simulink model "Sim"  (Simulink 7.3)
settings: Solver=ode45  StartTime=0.0  StopTime=30  MaxStep=0.01  RelTol=1e-3
InitFcn:
  | r2d=180/pi;
  | [Avn,Bvn,Cvn,Dvn]= Vehi_20flx;              % Load Nomin Inters. Stiff Vehi
  | [Avr,Bvr,Cvr,Dvr]= Vehi_20rif;              % Load Hard Interst. Stiff Vehi
  | [Avs,Bvs,Cvs,Dvs]= Vehi_20sif;              % Load Soft Interst. Stiff Vehi
  | [Aa,Ba,Ca,Da]= actuator;                    % Load Actuator system
  | 
  | zn=0.02; wn=7.4; zd=0.2; wd=7;              % Filter-1
  | zn2=0.015; wn2=16.8; zd2=0.2; wd2=16;       % Filter-2
  | %[Af,Bf,Cf,Df]= linmod('Actor'); sysf= SS(Af,Bf,Cf,Df);
  | Iy=2.163e8; T=2847083; l=113.6;
  | om=0.145*6.28; wf=9;
  | Kp=om^2*Iy/(l*T); Kr=2*0.85*om*Iy/(l*T);
  | 
  | Av2=Avs; Bv2=Bvs; Cv2=Cvs; Dv2=Dvs;       % Use the Nominal in the Simulat
StopFcn:
  | Pl
undefined symbols (not defined in the file or in its folder): Aa, Ba, Ca, Da

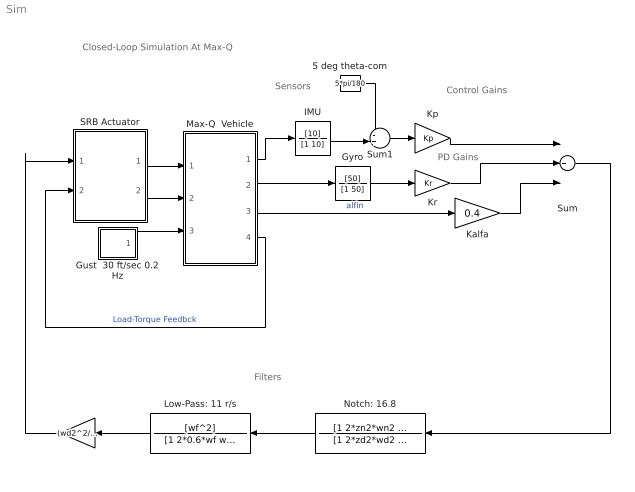
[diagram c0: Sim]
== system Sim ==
  note: Sensors
  note: PD Gains
  note: Filters
  note: Closed-Loop Simulation At Max-Q
  note: Control Gains
  "  " : Gain  Gain=(wd2^2/wn2^2)  ParameterDataType=sfix(16)  ParameterScaling=2^0  OutDataType=sfix(16)  OutScaling=2^0
  5 deg theta-com : Constant  Value=5*pi/180  OutDataType=sfix(16)  OutScaling=2^0
  Gust  30 ft/sec 0.2 Hz : Subsystem
  Gyro : TransferFcn  Numerator=[50]  Denominator=[1 50]
  IMU : TransferFcn  Numerator=[10]  Denominator=[1 10]
  Kalfa : Gain  Gain=0.4  ParameterDataType=sfix(16)  ParameterScaling=2^0  OutDataType=sfix(16)  OutScaling=2^0
  Kp : Gain  Gain=Kp  ParameterDataType=sfix(16)  ParameterScaling=2^0  OutDataType=sfix(16)  OutScaling=2^0
  Kr : Gain  Gain=Kr  ParameterDataType=sfix(16)  ParameterScaling=2^0  OutDataType=sfix(16)  OutScaling=2^0
  Low-Pass: 11 r/s : TransferFcn  Numerator=[wf^2]  Denominator=[1 2*0.6*wf wf^2]
  Max-Q  Vehicle : Subsystem
  Notch: 16.8 : TransferFcn  Numerator=[1 2*zn2*wn2 wn2^2]  Denominator=[1 2*zd2*wd2 wd2^2]
  SRB Actuator : Subsystem
  Sum : Sum  Inputs=+++  OutDataType=sfix(16)  OutScaling=2^0
  Sum1 : Sum  Inputs=-+|  OutDataType=sfix(16)  OutScaling=2^0
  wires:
  SRB Actuator/1(delto) -> Max-Q  Vehicle/1(delta)
  SRB Actuator/2(delt-dd) -> Max-Q  Vehicle/2(delt-dd)
  Max-Q  Vehicle/4(TL) -> SRB Actuator/2(Ld-Tq)  "Load-Torque Feedbck"
  Max-Q  Vehicle/3(alflex) -> Kalfa/1  "alfin"
  Kp/1 -> Sum/1
  Kr/1 -> Sum/2
  Max-Q  Vehicle/1(Theta) -> IMU/1
  Max-Q  Vehicle/2(q-flx) -> Gyro/1
  Sum/1 -> Notch: 16.8/1
  Gyro/1 -> Kr/1
  Low-Pass: 11 r/s/1 -> "  "/1
  Gust  30 ft/sec 0.2 Hz/1(Vgust) -> Max-Q  Vehicle/3(Gust)
  IMU/1 -> Sum1/2
  Sum1/1 -> Kp/1
  Kalfa/1 -> Sum/3
  Notch: 16.8/1 -> Low-Pass: 11 r/s/1
  "  "/1 -> SRB Actuator/1(delti)
  5 deg theta-com/1 -> Sum1/1

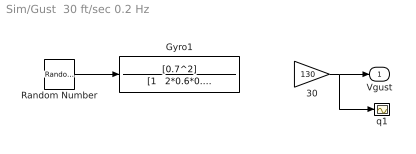
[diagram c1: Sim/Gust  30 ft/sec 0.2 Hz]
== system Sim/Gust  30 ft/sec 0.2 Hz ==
  30 : Gain  Gain=130  ParameterDataType=sfix(16)  ParameterScaling=2^0  OutDataType=sfix(16)  OutScaling=2^0
  Gyro1 : TransferFcn  Numerator=[0.7^2]  Denominator="[1   2*0.6*0.7   0.7^2]"
  Random Number : RandomNumber  Seed=-2  SampleTime=0
  q1 : Scope
  Vgust : Outport  OutDataType=sfix(16)  OutScaling=2^0
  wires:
  Random Number/1 -> Gyro1/1
  30/1 -> Vgust/1, q1/1

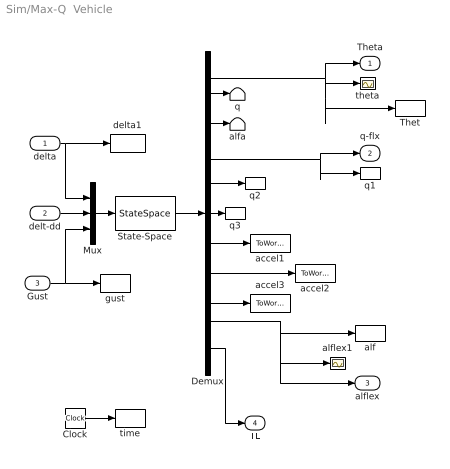
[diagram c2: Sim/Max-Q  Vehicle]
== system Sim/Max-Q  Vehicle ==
  delta : Inport  OutDataType=sfix(16)  OutScaling=2^0
  delt-dd : Inport  Port=2  OutDataType=sfix(16)  OutScaling=2^0
  Gust : Inport  Port=3  OutDataType=sfix(16)  OutScaling=2^0
  Clock : Clock
  Demux : Demux  Outputs=11
  Mux : Mux  Inputs=3
  State-Space : StateSpace  A=Av2  B=Bv2  C=Cv2  D=Dv2
  Thet : ToWorkspace  VariableName=theta  SampleTime=-1  SaveFormat=Array
  accel1 : ToWorkspace  VariableName=accel1  SampleTime=-1  SaveFormat=Array
  accel2 : ToWorkspace  VariableName=accel2  SampleTime=-1  SaveFormat=Array
  accel3 : ToWorkspace  VariableName=accel3  SampleTime=-1  SaveFormat=Array
  alf : ToWorkspace  VariableName=alpha  SampleTime=-1  SaveFormat=Array
  alfa : Terminator
  alflex1 : Scope
  delta1 : ToWorkspace  VariableName=delta  SampleTime=-1  SaveFormat=Array
  gust : ToWorkspace  VariableName=Gust  SampleTime=-1  SaveFormat=Array
  q : Terminator
  q1 : ToWorkspace  VariableName=q1  SampleTime=-1  SaveFormat=Array
  q2 : ToWorkspace  VariableName=q2  SampleTime=-1  SaveFormat=Array
  q3 : ToWorkspace  VariableName=q3  SampleTime=-1  SaveFormat=Array
  theta : Scope
  time : ToWorkspace  VariableName=time  SampleTime=-1  SaveFormat=Array
  Theta : Outport  OutDataType=sfix(16)  OutScaling=2^0
  q-flx : Outport  Port=2  OutDataType=sfix(16)  OutScaling=2^0
  alflex : Outport  Port=3  OutDataType=sfix(16)  OutScaling=2^0
  TL : Outport  Port=4  OutDataType=sfix(16)  OutScaling=2^0
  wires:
  Demux/7 -> accel1/1
  Demux/10 -> alflex/1, alflex1/1, alf/1
  Demux/3 -> alfa/1
  Demux/9 -> accel3/1
  Demux/6 -> q3/1
  State-Space/1 -> Demux/1
  Demux/11 -> TL/1
  Demux/5 -> q2/1
  Demux/2 -> q/1
  Demux/8 -> accel2/1
  Demux/4 -> q-flx/1, q1/1
  Demux/1 -> Theta/1, theta/1, Thet/1
  Gust/1 -> Mux/3, gust/1
  delt-dd/1 -> Mux/2
  delta/1 -> Mux/1, delta1/1
  Mux/1 -> State-Space/1
  Clock/1 -> time/1

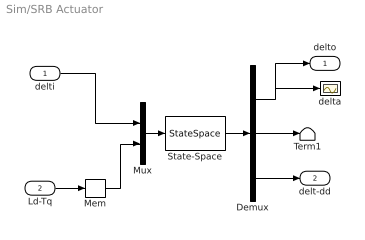
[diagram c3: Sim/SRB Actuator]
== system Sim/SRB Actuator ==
  delti : Inport  OutDataType=sfix(16)  OutScaling=2^0
  Ld-Tq : Inport  Port=2  OutDataType=sfix(16)  OutScaling=2^0
  Demux : Demux  Outputs=3
  Mem : Memory
  Mux : Mux  Inputs=2
  State-Space : StateSpace  A=Aa  B=Ba  C=Ca  D=Da
  Term1 : Terminator
  delta : Scope
  delto : Outport  OutDataType=sfix(16)  OutScaling=2^0
  delt-dd : Outport  Port=2  OutDataType=sfix(16)  OutScaling=2^0
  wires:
  Mux/1 -> State-Space/1
  State-Space/1 -> Demux/1
  Demux/1 -> delto/1, delta/1
  delti/1 -> Mux/1
  Ld-Tq/1 -> Mem/1
  Demux/3 -> delt-dd/1
  Demux/2 -> Term1/1
  Mem/1 -> Mux/2
